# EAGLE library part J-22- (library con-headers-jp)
HEADER JACK PINS
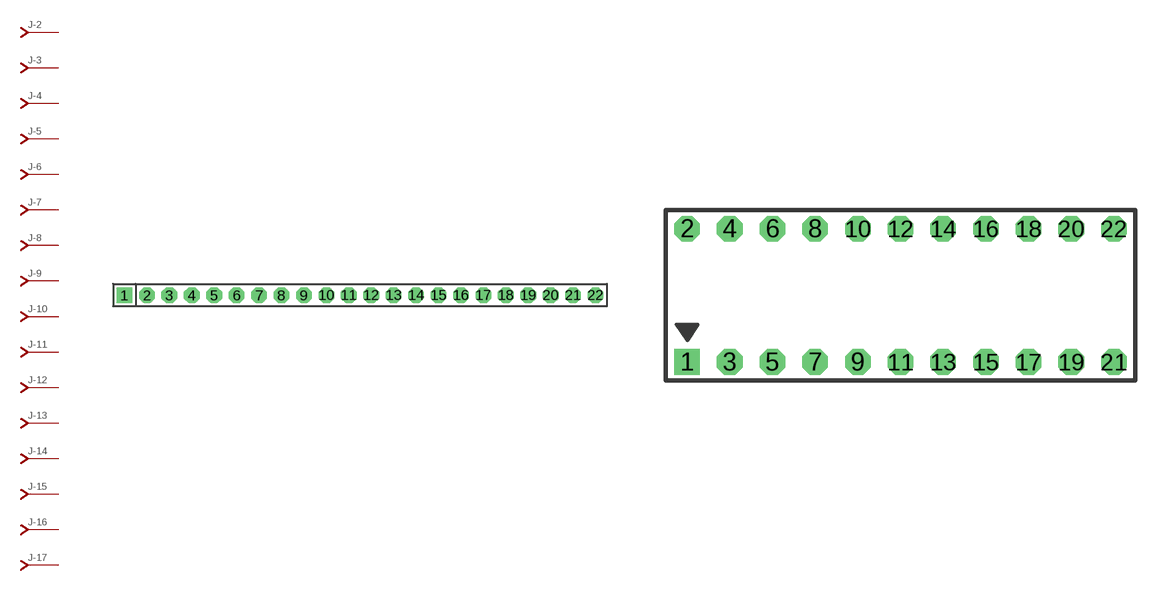
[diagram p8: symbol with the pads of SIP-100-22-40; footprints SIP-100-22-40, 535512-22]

Designator prefix J; gates -2=J-N -3=J-N -4=J-N -5=J-N -6=J-N -7=J-N -8=J-N -9=J-N -10=J-N -11=J-N -12=J-N -13=J-N -14=J-N -15=J-N -16=J-N -17=J-N -18=J-N -19=J-N -20=J-N -21=J-N -22=J-N -1=J-NV

## J-22-SIP-100-40  [SIP-100-22-40]
1  -1:J  pas
2  -2:J  pas
3  -3:J  pas
4  -4:J  pas
5  -5:J  pas
6  -6:J  pas
7  -7:J  pas
8  -8:J  pas
9  -9:J  pas
10  -10:J  pas
11  -11:J  pas
12  -12:J  pas
13  -13:J  pas
14  -14:J  pas
15  -15:J  pas
16  -16:J  pas
17  -17:J  pas
18  -18:J  pas
19  -19:J  pas
20  -20:J  pas
21  -21:J  pas
22  -22:J  pas

## J-22-535512  [535512-22]
Pads as for SIP-100-22-40

## J-22-79107  [79107-22]
Pads as for SIP-100-22-40

## J-22-79109  [79109-22]
Pads as for SIP-100-22-40

## J-22-87264  [87264-22]
Pads as for SIP-100-22-40

## J-22-87368  [87368-22]
Pads as for SIP-100-22-40

## J-22-100-2X11  [DIL-100-2X11]
Pads as for SIP-100-22-40

## J-22-100-2X11_M  [DIL-100-2X11_M]
Pads as for SIP-100-22-40

## J-22-2MM-2X11  [DIL-2MM-2X11]
Pads as for SIP-100-22-40

## J-22-2MM-2X11_M  [DIL-2MM-2X11_M]
Pads as for SIP-100-22-40

## J-22-SIP-100-32  [SIP-100-22-32]
Pads as for SIP-100-22-40

## J-22-SIP-100-40Y  [SIP-100-22-40Y]
Pads as for SIP-100-22-40

## J-22-SIP-100-32Y  [SIP-100-22-32Y]
Pads as for SIP-100-22-40

## J-22-71991  [71991-22]
Pads as for SIP-100-22-40

## J-22-KK-4455-B22  [KK-4455-B22]
Pads as for SIP-100-22-40

## J-22-KK-4455-A22  [KK-4455-A22]
Pads as for SIP-100-22-40

## J-22-KK-4455-C22  [KK-4455-C22]
Pads as for SIP-100-22-40

## Footprint SIP-100-22-40 (pad centres in mm)
SIP Header - 0.1", 40 mil drill
drill 1.016 pad 1.778 square: 1 -26.67,0
drill 1.016 pad 1.778 octagon: 2 -24.13,0; 3 -21.59,0; 4 -19.05,0; 5 -16.51,0; 6 -13.97,0; 7 -11.43,0; 8 -8.89,0; 9 -6.35,0; 10 -3.81,0; 11 -1.27,0; 12 1.27,0; 13 3.81,0; 14 6.35,0; 15 8.89,0; 16 11.43,0; 17 13.97,0; 18 16.51,0; 19 19.05,0; 20 21.59,0; 21 24.13,0; 22 26.67,0

## Footprint 535512-22 (pad centres in mm)
AMPMODU - 535512 Series
drill 1.016 square: 1 -12.7,0
drill 1.016 octagon: 2 -12.7,7.938; 3 -10.16,0; 4 -10.16,7.938; 5 -7.62,0; 6 -7.62,7.938; 7 -5.08,0; 8 -5.08,7.938; 9 -2.54,0; 10 -2.54,7.938; 11 0,0; 12 0,7.938; 13 2.54,0; 14 2.54,7.938; 15 5.08,0; 16 5.08,7.938; 17 7.62,0; 18 7.62,7.938; 19 10.16,0; 20 10.16,7.938; 21 12.7,0; 22 12.7,7.938

## Footprint 79107-22 (pad centres in mm)
Molex Board-To-Board Receptacal 2.00mm (.079") Pitch Milli-Grid Header, Vertical, Through-Hole Mates with: 87759, 87762, 87758, 87760
drill 0.711 square: 1 -10,-1
drill 0.711: 2 -10,1; 3 -8,-1; 4 -8,1; 5 -6,-1; 6 -6,1; 7 -4,-1; 8 -4,1; 9 -2,-1; 10 -2,1; 11 0,-1; 12 0,1; 13 2,-1; 14 2,1; 15 4,-1; 16 4,1; 17 6,-1; 18 6,1; 19 8,-1; 20 8,1; 21 10,-1; 22 10,1

## Footprint 79109-22 (pad centres in mm)
Molex Board-to-Board Receptacal 2.00mm (.079") Pitch Milli-Grid Header, Vertical, Top/Bottom Entry Mates with: 87758, 87759, 87760, 87831, 87832, 87833
smd 1.12 x 1.83: 1 -10,-2.65; 2 -10,2.65; 3 -8,-2.65; 4 -8,2.65; 5 -6,-2.65; 6 -6,2.65; 7 -4,-2.65; 8 -4,2.65; 9 -2,-2.65; 10 -2,2.65; 11 0,-2.65; 12 0,2.65; 13 2,-2.65; 14 2,2.65; 15 4,-2.65; 16 4,2.65; 17 6,-2.65; 18 6,2.65; 19 8,-2.65; 20 8,2.65; 21 10,-2.65; 22 10,2.65
hole 0.914 at -9,0
hole 0.914 at -10,1
hole 0.914 at -10,-1
hole 0.914 at -8,-1
hole 0.914 at -8,1
hole 0.914 at -6,-1
hole 0.914 at -6,1
hole 0.914 at 9,0
hole 0.914 at -4,1
hole 0.914 at -4,-1
hole 0.914 at -2,1
hole 0.914 at -2,-1
hole 0.914 at 0,1
hole 0.914 at 0,-1
hole 0.914 at 2,1
hole 0.914 at 2,-1
hole 0.914 at 4,-1
hole 0.914 at 4,1
hole 0.914 at 6,1
hole 0.914 at 6,-1
hole 0.914 at 8,1
hole 0.914 at 8,-1
hole 0.914 at 10,1
hole 0.914 at 10,-1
